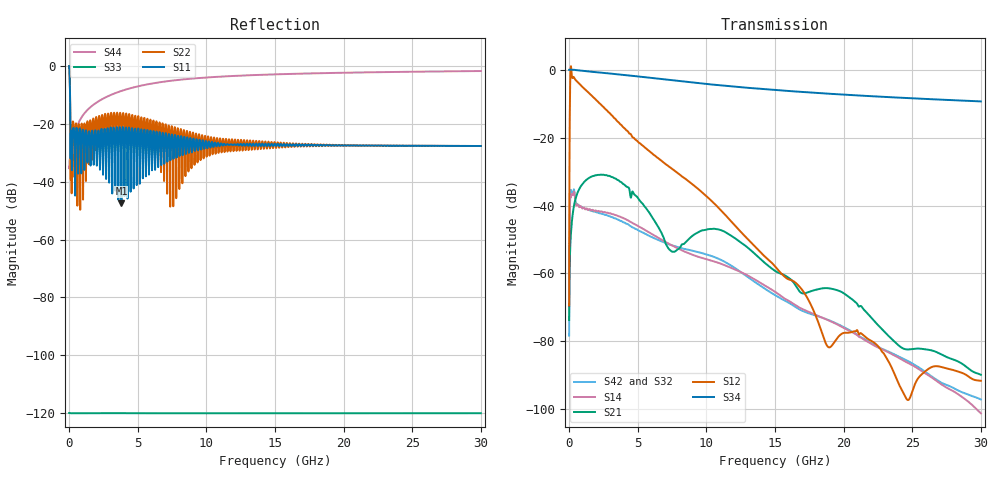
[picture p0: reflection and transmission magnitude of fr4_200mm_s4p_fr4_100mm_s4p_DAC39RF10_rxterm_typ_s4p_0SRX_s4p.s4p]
! Touchstone generated by fitter/viewer
# HZ S  RI R 5.000000e+01
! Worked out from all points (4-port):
!   3899 points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, 7.694 MHz to 30 GHz, reference 50 ohm
!   strongest paths, dB at 7.694 MHz, 7.502 GHz, 15 GHz, 22.51 GHz, 30 GHz:
!     S34: 0.2, -2.9, -5.8, -7.8, -9.2
!     S12: -69.5, -29.1, -57.9, -81.5, -91.8
!     S21: -73.8, -53.6, -59.3, -75.3, -90.0
!     S14: -72.5, -51.8, -65.5, -81.9, -101.4
!     S42: -78.5, -51.7, -66.4, -81.7, -97.3
!     S32: -78.5, -51.7, -66.4, -81.7, -97.3
!   lowest |S11| = -47.5 dB at 3.816 GHz (marker M1), VSWR 1.01, Z = 49.6 - j0.0314 ohm
!   |S11| at or under -10 dB: 75.75 MHz to end of sweep
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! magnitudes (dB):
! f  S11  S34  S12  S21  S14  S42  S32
! 7.694 MHz  -0.1  0.2  -69.5  -73.8  -72.5  -78.5  -78.5
! 230.8 MHz  -28.6  0.2  -2.2  -43.8  -36.6  -36.8  -36.8
! 3.816 GHz  -47.5  -1.3  -16.2  -33.1  -43.5  -44.6  -44.6
! 7.471 GHz  -24.1  -2.9  -29.0  -53.5  -51.7  -51.7  -51.7
! 10.88 GHz  -26.7  -4.4  -40.6  -47.0  -56.9  -55.7  -55.7
! 18.71 GHz  -27.5  -6.9  -80.8  -64.4  -73.6  -73.5  -73.5
! 30 GHz  -27.7  -9.2  -91.8  -90.0  -101.4  -97.3  -97.3
